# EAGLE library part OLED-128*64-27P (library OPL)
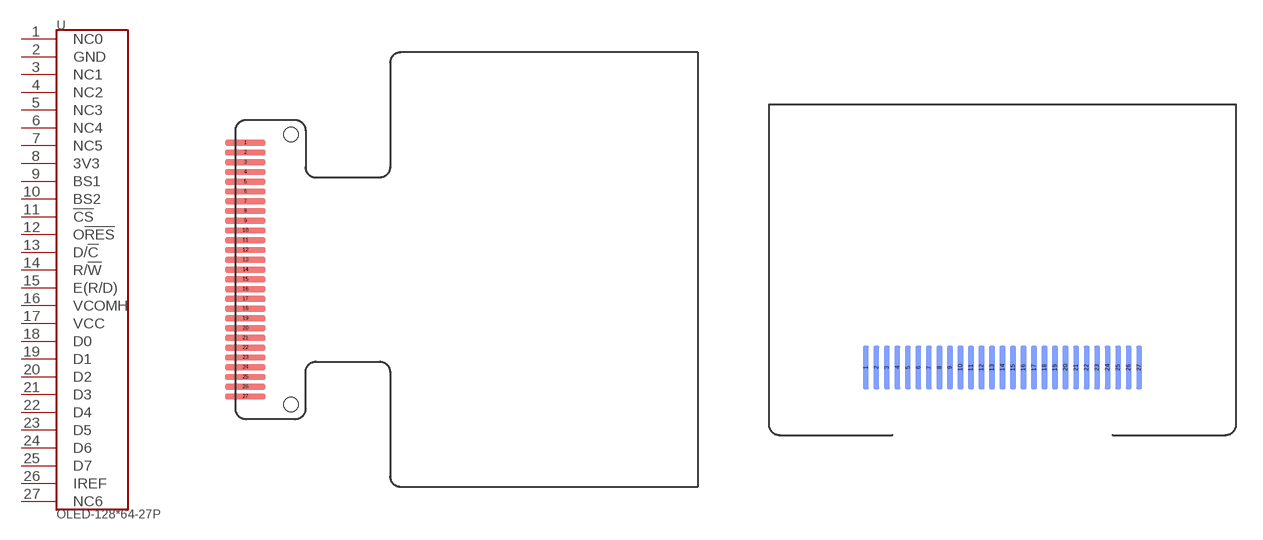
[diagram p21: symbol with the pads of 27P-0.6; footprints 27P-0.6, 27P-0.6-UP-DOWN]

Designator prefix U

## OLED-12864-27P-308020000-F  [27P-0.6]
1  NC0
2  GND
3  NC1
4  NC2
5  NC3
6  NC4
7  NC5
8  3V3
9  BS1
10  BS2
11  !CS
12  O!RES
13  D/!C
14  R/!W
15  E(R/D)
16  VCOMH
17  VCC
18  D0
19  D1
20  D2
21  D3
22  D4
23  D5
24  D6
25  D7
26  IREF
27  NC6

## OLED-12864-27P-308020000-U  [27P-0.6-UP-DOWN]
Pads as for 27P-0.6

## OLED-12864-27P-308020000-BEND  [27P-0.6-BEND]
Pads as for 27P-0.6

## Footprint 27P-0.6 (pad centres in mm)
smd 2.5 x 0.35: 1 0.6,7.8; 2 0.6,7.2; 3 0.6,6.6; 4 0.6,6; 5 0.6,5.4; 6 0.6,4.8; 7 0.6,4.2; 8 0.6,3.6; 9 0.6,3; 10 0.6,2.4; 11 0.6,1.8; 12 0.6,1.2; 13 0.6,0.6; 14 0.6,0; 15 0.6,-0.6; 16 0.6,-1.2; 17 0.6,-1.8; 18 0.6,-2.4; 19 0.6,-3; 20 0.6,-3.6; 21 0.6,-4.2; 22 0.6,-4.8; 23 0.6,-5.4; 24 0.6,-6; 25 0.6,-6.6; 26 0.6,-7.2; 27 0.6,-7.8
hole 0.889 at 3.4,8.3
hole 0.889 at 3.4,-8.3

## Footprint 27P-0.6-UP-DOWN (pad centres in mm)
smd 0.35 x 2.5 bottom: 1 -7.8,-3.14; 2 -7.2,-3.14; 3 -6.6,-3.14; 4 -6,-3.14; 5 -5.4,-3.14; 6 -4.8,-3.14; 7 -4.2,-3.14; 8 -3.6,-3.14; 9 -3,-3.14; 10 -2.4,-3.14; 11 -1.8,-3.14; 12 -1.2,-3.14; 13 -0.6,-3.14; 14 0,-3.14; 15 0.6,-3.14; 16 1.2,-3.14; 17 1.8,-3.14; 18 2.4,-3.14; 19 3,-3.14; 20 3.6,-3.14; 21 4.2,-3.14; 22 4.8,-3.14; 23 5.4,-3.14; 24 6,-3.14; 25 6.6,-3.14; 26 7.2,-3.14; 27 7.8,-3.14

## Footprint 27P-0.6-BEND (pad centres in mm)
smd 0.35 x 2.5: 1 -7.805,5.624; 2 -7.205,5.624; 3 -6.605,5.624; 4 -6.005,5.624; 5 -5.405,5.624; 6 -4.805,5.624; 7 -4.205,5.624; 8 -3.605,5.624; 9 -3.005,5.624; 10 -2.405,5.624; 11 -1.805,5.624; 12 -1.205,5.624; 13 -0.605,5.624; 14 -0.005,5.624; 15 0.595,5.624; 16 1.195,5.624; 17 1.795,5.624; 18 2.395,5.624; 19 2.995,5.624; 20 3.595,5.624; 21 4.195,5.624; 22 4.795,5.624; 23 5.395,5.624; 24 5.995,5.624; 25 6.595,5.624; 26 7.195,5.624; 27 7.795,5.624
